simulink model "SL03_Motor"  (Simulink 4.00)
settings: Solver=ode45  StartTime=0.0  StopTime=300.0  RelTol=1e-3
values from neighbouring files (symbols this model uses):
  A = [ -R/L, -k/L; k/J, -h/J ]    [SL03_MotorAnalysis.m]    (also in SL03_MotorParameters.m)
  B = [ 1/L, 0; 0, -1/J ]    [SL03_MotorAnalysis.m]    (also in SL03_MotorParameters.m)
  C = [ 0 1 ]    [SL03_MotorAnalysis.m]    (also in SL03_MotorParameters.m)
  D = [ 0 0 ]    [SL03_MotorAnalysis.m]    (also in SL03_MotorParameters.m)
libraries: simulink3 x1

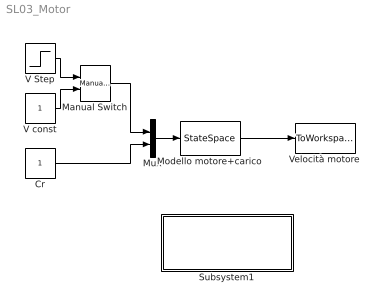
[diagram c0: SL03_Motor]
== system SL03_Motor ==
  Cr : Constant  Value=1
  Manual Switch : simulink3/Nonlinear/Manual Switch  sw=1  action=0
  Modello motore+carico : StateSpace  A=A  B=B  C=C  D=D  X0=[ 0 0 ]  Realization=auto  AbsoluteTolerance=auto
  Mux : Mux  Inputs=2
  Subsystem1 : Subsystem
  V Step : Step  Time=1  Before=0  After=220  SampleTime=0
  V const : Constant  Value=1
  Velocità motore : ToWorkspace  VariableName=w  SampleTime=-1  SaveFormat=Array
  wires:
  Mux/1 -> Modello motore+carico/1
  Modello motore+carico/1 -> Velocità motore/1
  Cr/1 -> Mux/2
  Manual Switch/1 -> Mux/1
  V const/1 -> Manual Switch/2
  V Step/1 -> Manual Switch/1

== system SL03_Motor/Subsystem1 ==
